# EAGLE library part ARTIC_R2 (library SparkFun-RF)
AnSem ARTIC R2 Chipset The ARTIC is an integrated low power small size ARGOS 2/3/4 single chip radio. ARTIC implements a message based wireless interface. For satellite uplink communication, ARTIC will encode, modulate and transmit provided user messages. For downlink communication, ARTIC will lock to the downstream, demodulate and decode and extract the satellite messages. The ARTIC can transmit signals in frequency bands around 400MHz and receive signals in the bands around 466MHz, in accordance with the ARGOS satellite system specifications. The ARTIC is compliant and certified for all ARGOS 2 and ARGOS 3 TX standards. It contains a RF transceiver, afrequency synthesizer and a digital baseband modem. The ARTIC contains an on-chip power amplifier delivering 1mW [0dBm] output power, that serves as an output for connecting an external high efficient PA. The (de)modulation algorithms run on an on-chip DSP. This software approach allows for retargeting the ARTIC for other applications. The DSP program can be retained on an external flash or the MCU.
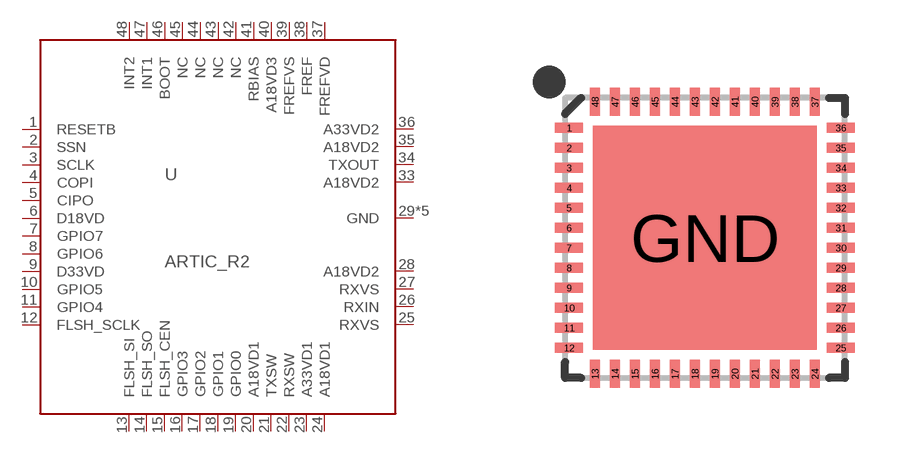
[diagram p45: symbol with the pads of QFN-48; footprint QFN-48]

Designator prefix U

## ARTIC_R2 (PROD_ID: IC-15312)  [QFN-48]
1  RESETB
2  SSN
3  SCLK
4  COPI
5  CIPO
6  D18VD  pwr
7  GPIO7
8  GPIO6
9  D33VD  pwr
10  GPIO5
11  GPIO4
12  FLSH_SCLK
13  FLSH_SI
14  FLSH_SO
15  FLSH_CEN
16  GPIO3
17  GPIO2
18  GPIO1
19  GPIO0
20  A18VD1  pwr
21  TXSW
22  RXSW
23  A33VD1  pwr
24  A18VD1  pwr
25  RXVS
26  RXIN
27  RXVS
28  A18VD2  pwr
29  GND
30  GND
31  GND
32  GND
33  A18VD2  pwr
34  TXOUT
35  A18VD2  pwr
36  A33VD2  pwr
37  FREFVD
38  FREF
39  FREFVS
40  A18VD3  pwr
41  RBIAS
42  NC  nc
43  NC  nc
44  NC  nc
45  NC  nc
46  BOOT
47  INT1
48  INT2
GND  GND

## Footprint QFN-48 (pad centres in mm)
48-pin QFN (7x7mm, 0.5mm pitch)
smd 0.7 x 0.25: 1 -3.4,2.75; 2 -3.4,2.25; 3 -3.4,1.75; 4 -3.4,1.25; 5 -3.4,0.75; 6 -3.4,0.25; 7 -3.4,-0.25; 8 -3.4,-0.75; 9 -3.4,-1.25; 10 -3.4,-1.75; 11 -3.4,-2.25; 12 -3.4,-2.75; 25 3.4,-2.75; 26 3.4,-2.25; 27 3.4,-1.75; 28 3.4,-1.25; 29 3.4,-0.75; 30 3.4,-0.25; 31 3.4,0.25; 32 3.4,0.75; 33 3.4,1.25; 34 3.4,1.75; 35 3.4,2.25; 36 3.4,2.75
smd 0.25 x 0.7: 13 -2.75,-3.4; 14 -2.25,-3.4; 15 -1.75,-3.4; 16 -1.25,-3.4; 17 -0.75,-3.4; 18 -0.25,-3.4; 19 0.25,-3.4; 20 0.75,-3.4; 21 1.25,-3.4; 22 1.75,-3.4; 23 2.25,-3.4; 24 2.75,-3.4; 37 2.75,3.4; 38 2.25,3.4; 39 1.75,3.4; 40 1.25,3.4; 41 0.75,3.4; 42 0.25,3.4; 43 -0.25,3.4; 44 -0.75,3.4; 45 -1.25,3.4; 46 -1.75,3.4; 47 -2.25,3.4; 48 -2.75,3.4
smd 5.6 x 5.6: GND 0,0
